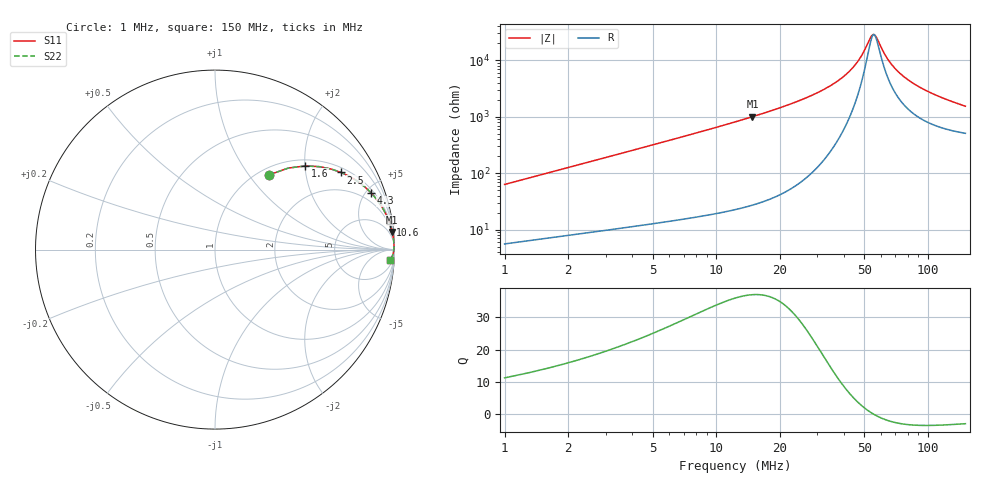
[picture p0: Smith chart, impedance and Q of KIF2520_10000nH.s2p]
!version-2
!date-12.2020
!Series
# MHz S RI R 50
!Freq ReS11 ImS11 ReS21 ImS21 ReS12 ImS12 ReS22 ImS22
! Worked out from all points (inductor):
!   498 points, 1 MHz to 150 MHz, reference 50 ohm
!   read as one part in series: L = 10 uH near 1.6 MHz
!   highest Q = 37 at 14.8 MHz (marker M1), where L = 10.8 uH
!   self-resonance near 55.3 MHz
!   S11 on the Smith chart (normalised r, x): 1 MHz: 1.11, +1.26; 1.6 MHz: 1.14, +2.01; 2.5 MHz: 1.18, +3.15; 4.3 MHz: 1.23, +5.44; 10.6 MHz: 1, +14; 150 MHz: 11, -29
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1  0.3006 0.4164  0.6994 -0.4164  0.6994 -0.4164  0.3006 0.4164
1.6  0.504 0.4662  0.496 -0.4662  0.496 -0.4662  0.504 0.4662
2.5  0.7028 0.4298  0.2972 -0.4298  0.2972 -0.4298  0.7028 0.4298
3.4  0.8103 0.3687  0.1897 -0.3687  0.1897 -0.3687  0.8103 0.3687
4.3  0.8707 0.3147  0.1293 -0.3147  0.1293 -0.3147  0.8707 0.3147
7  0.9459 0.2098  0.0541 -0.2098  0.0541 -0.2098  0.9459 0.2098
10.6  0.9756 0.1404  0.0244 -0.1404  0.0244 -0.1404  0.9756 0.1404
14.8  0.9875 0.0983  0.0125 -0.0983  0.0125 -0.0983  0.9875 0.0983
25.9  0.996 0.0477  0.00404 -0.0477  0.00404 -0.0477  0.996 0.0477
41.8  0.9974 0.0163  0.00258 -0.0163  0.00258 -0.0163  0.9974 0.0163
46.6  0.9972 0.01  0.00276 -0.01  0.00276 -0.01  0.9972 0.01
50.8  0.997 0.00507  0.00305 -0.00507  0.00305 -0.00507  0.997 0.00507
54.1  0.9967 0.00151  0.00334 -0.00151  0.00334 -0.00151  0.9967 0.00151
55.9  0.9965 -0.000329  0.00351 0.000329  0.00351 0.000329  0.9965 -0.000329
61.6  0.9958 -0.00577  0.00417 0.00577  0.00417 0.00577  0.9958 -0.00577
64.9  0.9954 -0.00869  0.00461 0.00869  0.00461 0.00869  0.9954 -0.00869
69.7  0.9947 -0.0127  0.0053 0.0127  0.0053 0.0127  0.9947 -0.0127
75.7  0.9937 -0.0174  0.00627 0.0174  0.00627 0.0174  0.9937 -0.0174
86.5  0.9917 -0.025  0.00826 0.025  0.00826 0.025  0.9917 -0.025
100.6  0.9887 -0.0339  0.0113 0.0339  0.0113 0.0339  0.9887 -0.0339
125.2  0.9826 -0.0472  0.0174 0.0472  0.0174 0.0472  0.9826 -0.0472
150  0.9755 -0.0585  0.0245 0.0585  0.0245 0.0585  0.9755 -0.0585
